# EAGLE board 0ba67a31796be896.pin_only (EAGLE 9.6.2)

Size 35 x 35 mm. Coordinates in mm from the lower left corner, seen from the top.
Outline: 0,3 0,32 arc-90 3,35 32,35 arc-90 35,32 35,3 arc-90 32,0 3,0 arc-90 0,3
Copper layers (1*16): Top 0.035mm / dielectric 1.5mm / Bottom 0.035mm
Design rules "PCBCart-Standard": minimum track width 8mil, minimum drill 0.4mm, track to track 8mil, track to pad 8mil, pad to pad 8mil, via to via 8mil, smd to smd 8mil, copper to edge 20mil, drill to drill 8mil, minimum pad ring 8mil, minimum via ring 10mil, stop-mask expansion 3mil, vias tented up to drill 20mil, thermal gap 8mil
tRestrict: area 19.1,21.6 to 19.6,21.7; area 22.1,21.6 to 22.6,21.7; area 22.1,22.1 to 22.7,22.4
bRestrict: area 26.5,31.5 to 26.7,32; area 30.7,13.6 to 31.2,13.7; area 30.7,15.4 to 31.2,15.5; area 31,23.7 to 31.5,23.9; area 31,25.4 to 31.5,25.5; area 28.3,31.5 to 28.4,32; area 3.2,12.2 to 3.3,12.7; area 1.1,12.2 to 1.3,12.7; area 5.7,12.2 to 5.8,12.7; area 3.7,12.2 to 3.8,12.7

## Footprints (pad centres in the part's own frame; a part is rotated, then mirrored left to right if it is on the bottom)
0805 = smd 1.3 x 1.5: 1 -0.95,0; 2 0.95,0
USB-MINIB_LARGER = smd 0.5 x 2.308: D+ 0,4.064; D- -0.8,4.064; GND 1.6,4.064; ID 0.8,4.064; VBUS -1.6,4.064 | smd 2.54 x 3.81: GND1 -4.4,-2; GND4 4.4,-2 | smd 2 x 2.4: GND2 -4.4,3.5; GND3 4.4,3.5 | hole 1: -2.2,1; 2.2,1
JSTPH2 = smd 1 x 4.6: 1 -1,-3.7; 2 1,-3.7 | smd 1.6 x 3.4: NC1 -3.4,1.5; NC2 3.4,1.5
1X02_OVAL = drill 1 long: 1 -1.27,0; 2 1.27,0
FIDUCIAL-1X2.5 = smd 1 x 1: 1 0,0
CHIPLED_0805 = smd 1.2 x 1.2: A 0,-1.05; C 0,1.05
0805-THM = drill 0.813 pad 1.676 octagon: 1 -5.08,0; 2 5.08,0
R0805 = smd 1.1 x 1.4: 1 -1,0; 2 1,0
DFN10_3X3MM = smd 2.35 x 1.58: GND 0,0 | smd 0.25 x 0.8: P$1 -1,-1.5; P$2 -0.5,-1.5; P$3 0,-1.5; P$4 0.5,-1.5; P$5 1,-1.5; P$6 1,1.5; P$7 0.5,1.5; P$8 0,1.5; P$9 -0.5,1.5; P$10 -1,1.5
MOUNTINGHOLE_2.0_PLATED = drill 2 pad 3: P$1 0,0

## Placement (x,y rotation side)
C1  10uF  [0805]  25.43,22.88 90 top
C2  10uF  [0805]  15.97,22.08 270 top
CN1  USB  [USB-MINIB_LARGER]  17.5,30.25 180 top
CN2  BATT_IN_JST  [JSTPH2]  24.51,3.81 180 top
CN3  LOAD_JST  [JSTPH2]  10.29,3.81 180 top
JP1  PWR_IN_0.1  [1X02_OVAL]  26.16,31.75 180 top
JP2  FIDUCIAL1.5X3  [FIDUCIAL-1X2.5]  8,26 0 top
JP3  LOAD_0.1  [1X02_OVAL]  31.24,23.37 270 top
JP4  FIDUCIAL1.5X3  [FIDUCIAL-1X2.5]  32,7 0 top
JP5  BATT_IN_0.1  [1X02_OVAL]  31.24,13.21 270 top
JP6  STAT  [1X02_OVAL]  31.24,18.29 270 top
LED1  STAT1-ORANGE  [CHIPLED_0805]  18.8,2.54 0 top
LED2  STAT2-GREEN  [CHIPLED_0805]  16.26,2.54 0 top
LED3  Power-RED  [CHIPLED_0805]  8.16,32.66 270 top
R1  150  [0805]  18.8,11.68 270 top
R2  150  [0805]  16.26,11.68 270 top
R3  150  [0805]  8.16,28.94 180 top
R4  PROG  [0805-THM]  4.7,17.53 90 top
R7  10K/THERM  [0805-THM]  2.16,17.53 90 top
RT1  1K  [R0805]  8.64,16.51 180 top
RT2  150K  [R0805]  8.64,18.8 180 top
U1  MCP73833T-AMI/MF  [DFN10_3X3MM]  20.81,20.86 270 top
U$11  MOUNTINGHOLE2.0  [MOUNTINGHOLE_2.0_PLATED]  32,3 0 top
U$14  [ADAFRUIT200MIL]  28.32,3.05 270 bottom
U$16  MOUNTINGHOLE2.0  [MOUNTINGHOLE_2.0_PLATED]  32,32 0 top
U$18  MOUNTINGHOLE2.0  [MOUNTINGHOLE_2.0_PLATED]  3,32 0 top
U$19  MOUNTINGHOLE2.0  [MOUNTINGHOLE_2.0_PLATED]  3,3 0 top

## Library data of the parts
C1 C2 CN1-CN3 JP1-JP6 LED1-LED3 R1-R4 U1 U$11 U$16 U$18 U$19 = microbuilder
R7 RT1 RT2 U$14 = adafruit

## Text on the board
tPlace: PWR | + | - | DCIN | THERM | PROG | - | BATT | + | RT2 | 1 | STAT | 2 | RT1 | - | BATT | LOAD | LOAD | + | DONE | CHRG
bPlace: MCP73833 LIPO/Li-Ion | Charger (3.7/4.2V) | 6V Max | DC IN: | 1000/PROG | CHRG RATE: | 1.0K=1000mA | 2.0K=500mA | 5.0K=200mA | Adafruit Industries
